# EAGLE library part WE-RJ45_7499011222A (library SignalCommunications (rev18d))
Order Code 7499011222A Design THT xBase-T 10/100 Base-T Ports 1x1 Application Standard Tab Position DOWN LED (Left-Right) Green-Green EMI Fingers Yes Details see: http://katalog.we-online.de/en/pbs/WE-LAN_RJ45/7499011222A? Updated by Yingchun Shan 2016-08-29 2016(C) Würth Elektronik
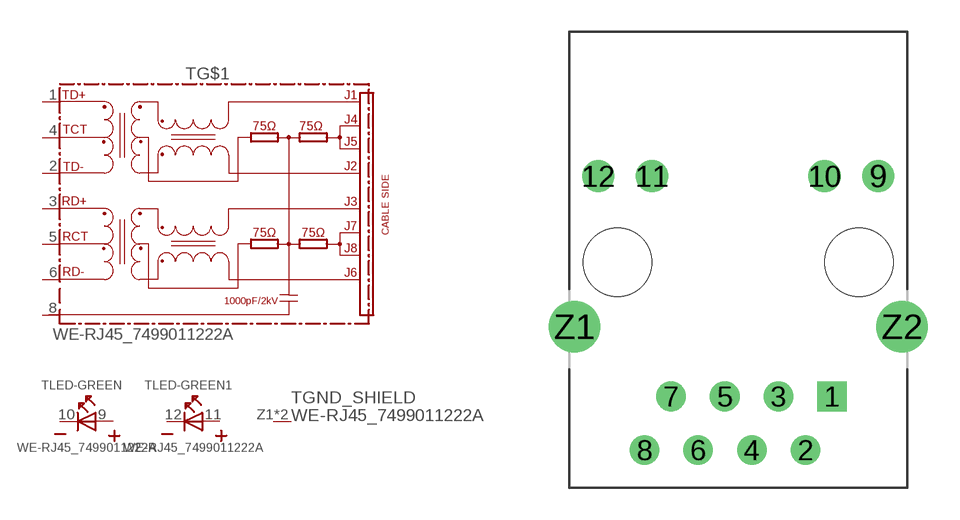
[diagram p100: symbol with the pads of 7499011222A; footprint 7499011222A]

Designator prefix T; gates LED-GREEN=LED2PIN LED-GREEN1=LED2PIN GND_SHIELD=GND_PIN G$1=74990X-THT-10/100-T

## WE-RJ45_7499011222A  [7499011222A]
1  G$1:TD+
2  G$1:TD-
3  G$1:RD+
4  G$1:TCT
5  G$1:RCT
6  G$1:RD-
8  G$1:8
9  LED-GREEN:A  pas
10  LED-GREEN:K  pas
11  LED-GREEN1:A  pas
12  LED-GREEN1:K  pas
Z1  GND_SHIELD:1  pwr
Z2  GND_SHIELD:1  pwr

## Footprint 7499011222A (pad centres in mm)
drill 0.89 square: 1 4.44,-6.35
drill 0.89: 2 3.18,-8.89; 3 1.9,-6.35; 4 0.64,-8.89; 5 -0.64,-6.35; 6 -1.9,-8.89; 7 -3.18,-6.35; 8 -4.44,-8.89
drill 1.02: 9 6.625,4.08; 10 4.085,4.08; 11 -4.085,4.08; 12 -6.625,4.08
drill 1.63: Z1 -7.745,-3.05; Z2 7.745,-3.05
hole 3.25 at 5.715,0
hole 3.25 at -5.715,0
